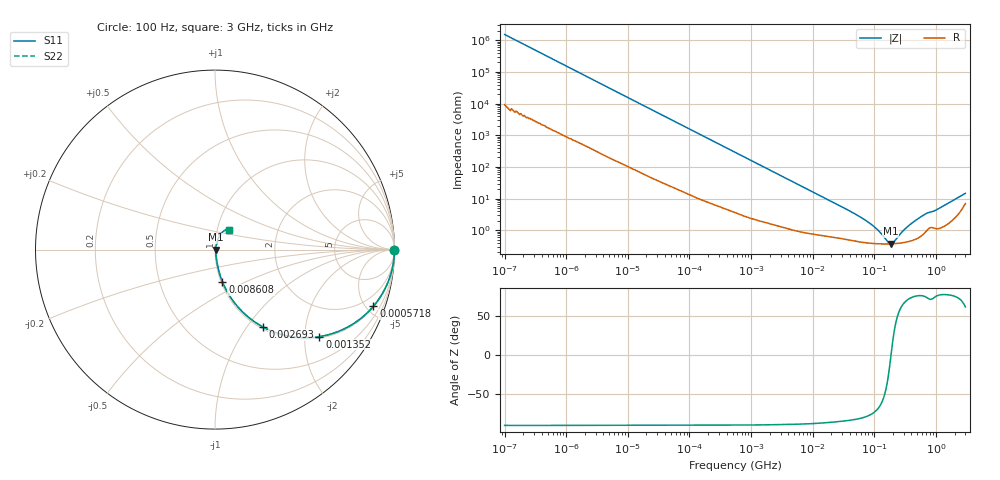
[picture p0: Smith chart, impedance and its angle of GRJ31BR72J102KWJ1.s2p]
!Murata Part Number: GRJ31BR72J102KWJ1
!These Parameters are Measured in Series Mode Connection
!Data Generated on Jun 19, 2026
!  o--ll--o
!Port1  Port2
!  o------o
!Operation Temp=25[degC], DC Bias Voltage=0[V]
!Freq. Start=100[Hz] Stop=3[GHz] 401[Steps]
# Hz S RI R 50
!Freq.(Hz) S11(Real) S11(Imag) S21(Real) S21(Imag) S12(Real) S12(Imag) S22(Real) S22(Imag)
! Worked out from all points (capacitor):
!   401 points, 100 Hz to 3 GHz, reference 50 ohm
!   read as one part in series: C = 1.04 nF near 109 Hz
!   lowest |Z| = 376 mohm at 182.8 MHz (marker M1)
!   series resonance near 186.2 MHz, so ESL is about 700 pH
!   S11 on the Smith chart (normalised r, x): 100 Hz: open; 571.8 kHz: 1.07, -5.56; 1.352 MHz: 1.04, -2.37; 2.693 MHz: 1.03, -1.20; 8.608 MHz: 1.02, -0.38; 3 GHz: 1.14, +0.26
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100  1 -6.53e-05  4e-07 6.53e-05  4e-07 6.53e-05  1 -6.53e-05
168  1 -0.000109  6e-07 0.000109  6e-07 0.000109  1 -0.000109
1788  1 -0.00116  8.4e-06 0.00116  8.4e-06 0.00116  1 -0.00116
31977  0.9994 -0.0204  0.000564 0.0204  0.000564 0.0204  0.9994 -0.0204
164120  0.9884 -0.1027  0.0116 0.1027  0.0116 0.1027  0.9884 -0.1027
547723  0.891 -0.3055  0.109 0.3055  0.109 0.3055  0.891 -0.3055
571812  0.8825 -0.3158  0.1175 0.3158  0.1175 0.3158  0.8825 -0.3158
879390  0.7638 -0.4177  0.2362 0.4177  0.2362 0.4177  0.7638 -0.4177
1352413  0.5819 -0.4849  0.4181 0.4849  0.4181 0.4849  0.5819 -0.4849
2692740  0.2682 -0.4316  0.7318 0.4316  0.7318 0.4316  0.2682 -0.4316
4513443  0.1211 -0.312  0.8789 0.312  0.8789 0.312  0.1211 -0.312
8607956  0.0416 -0.1798  0.9584 0.1798  0.9584 0.1798  0.0416 -0.1798
9794414  0.0339 -0.1595  0.9661 0.1595  0.9661 0.1595  0.0339 -0.1595
2.21892e7  0.0113 -0.0726  0.9887 0.0726  0.9887 0.0726  0.0113 -0.0726
7.093284e7  0.00447 -0.0205  0.9955 0.0205  0.9955 0.0205  0.00447 -0.0205
1.090876e8  0.00387 -0.0103  0.9961 0.0103  0.9961 0.0103  0.00387 -0.0103
1.751444e8  0.00373 -0.00113  0.9963 0.00113  0.9963 0.00113  0.00373 -0.00113
1.828475e8  0.00374 -0.000336  0.9963 0.000336  0.9963 0.000336  0.00374 -0.000336
2.080499e8  0.00379 0.00206  0.9962 -0.00206  0.9962 -0.00206  0.00379 0.00206
3.487234e8  0.00449 0.0125  0.9955 -0.0125  0.9955 -0.0125  0.00449 0.0125
5.59889e8  0.00694 0.0251  0.9931 -0.0251  0.9931 -0.0251  0.00694 0.0251
3e9  0.0787 0.111  0.9213 -0.111  0.9213 -0.111  0.0787 0.111
